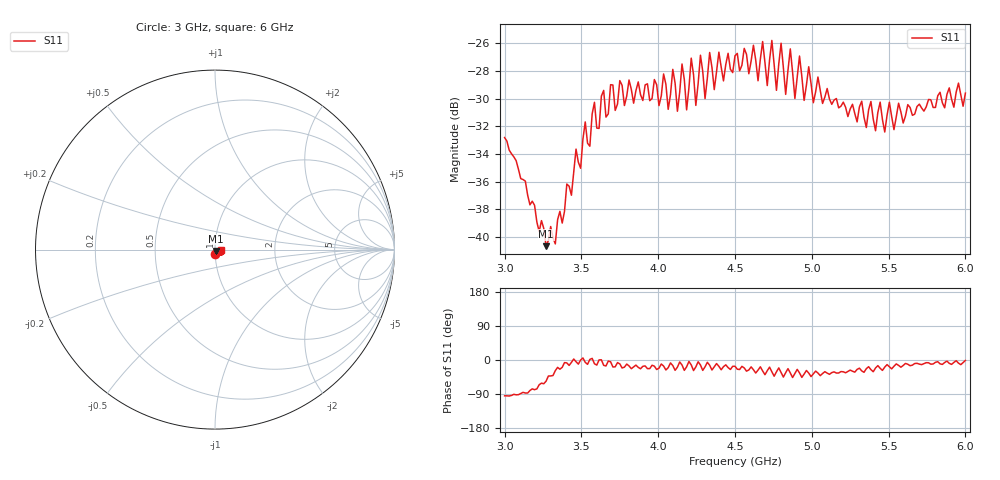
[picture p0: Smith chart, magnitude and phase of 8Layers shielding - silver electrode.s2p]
!  03/07/2025  16:54:27
! Ref Plane: 0.000 mm
# MHZ S MA R  50
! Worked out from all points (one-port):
!   201 points, 3 GHz to 6 GHz, reference 50 ohm
!   lowest |S11| = -40.7 dB at 3.27 GHz (marker M1), VSWR 1.02, Z = 50.5 - j0.776 ohm
!   |S11| at or under -10 dB: start of sweep to end of sweep
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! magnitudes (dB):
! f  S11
! 3 GHz  -32.8
! 3.27 GHz  -40.7
! 3.375 GHz  -39.0
! 3.525 GHz  -31.7
! 3.555 GHz  -33.4
! 3.585 GHz  -30.3
! 3.615 GHz  -32.1
! 3.75 GHz  -28.7
! 4.005 GHz  -30.5
! 4.035 GHz  -28.2
! 4.065 GHz  -30.8
! 4.095 GHz  -27.9
! 4.125 GHz  -30.9
! 4.155 GHz  -27.5
! 4.185 GHz  -30.8
! 4.215 GHz  -27.1
! 4.245 GHz  -30.5
! 4.275 GHz  -26.9
! 4.305 GHz  -30.0
! 4.335 GHz  -26.7
! 4.365 GHz  -29.3
! 4.395 GHz  -26.6
! 4.425 GHz  -28.7
! 4.5 GHz  -26.9
! 4.875 GHz  -28.1
! 5.25 GHz  -30.7
! 5.625 GHz  -30.4
! 6 GHz  -29.6
